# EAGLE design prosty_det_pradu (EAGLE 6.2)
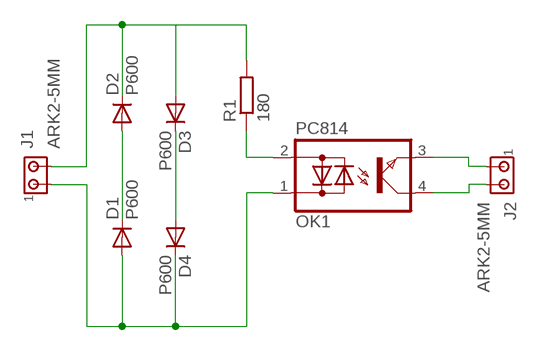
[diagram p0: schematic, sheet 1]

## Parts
D1  P600  [P6-15]
D2  P600  [P6-15]
D3  P600  [P6-15]
D4  P600  [P6-15]
J1  ARK2-5MM  [2PIN-5MM]
J2  ARK2-5MM  [2PIN-5MM]
OK1  PC814  [DIL04]
R1  180  R-EU_0207/7  [0207/7]

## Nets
N$1: D2.C D3.A J1.P$2 R1.2
N$2: D1.C D2.A
N$3: D3.C D4.A
N$5: J2.P$1 OK1.3(E)
N$6: J2.P$2 OK1.4(C)
N$7: D1.A D4.C J1.P$1 OK1.1(AC1)
N$8: OK1.2(AC2) R1.1

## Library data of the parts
D1-D4 = diode:P600: DIODE
J1 J2 = zlacza_futrzak:ARK2: ARK 2
OK1 = optocoupler:PC814: SHARP OPTO COUPLER; OC_FARNELL: 9707662; OC_NEWARK: unknown
R1 = rcl:R-EU_: RESISTOR, European symbol

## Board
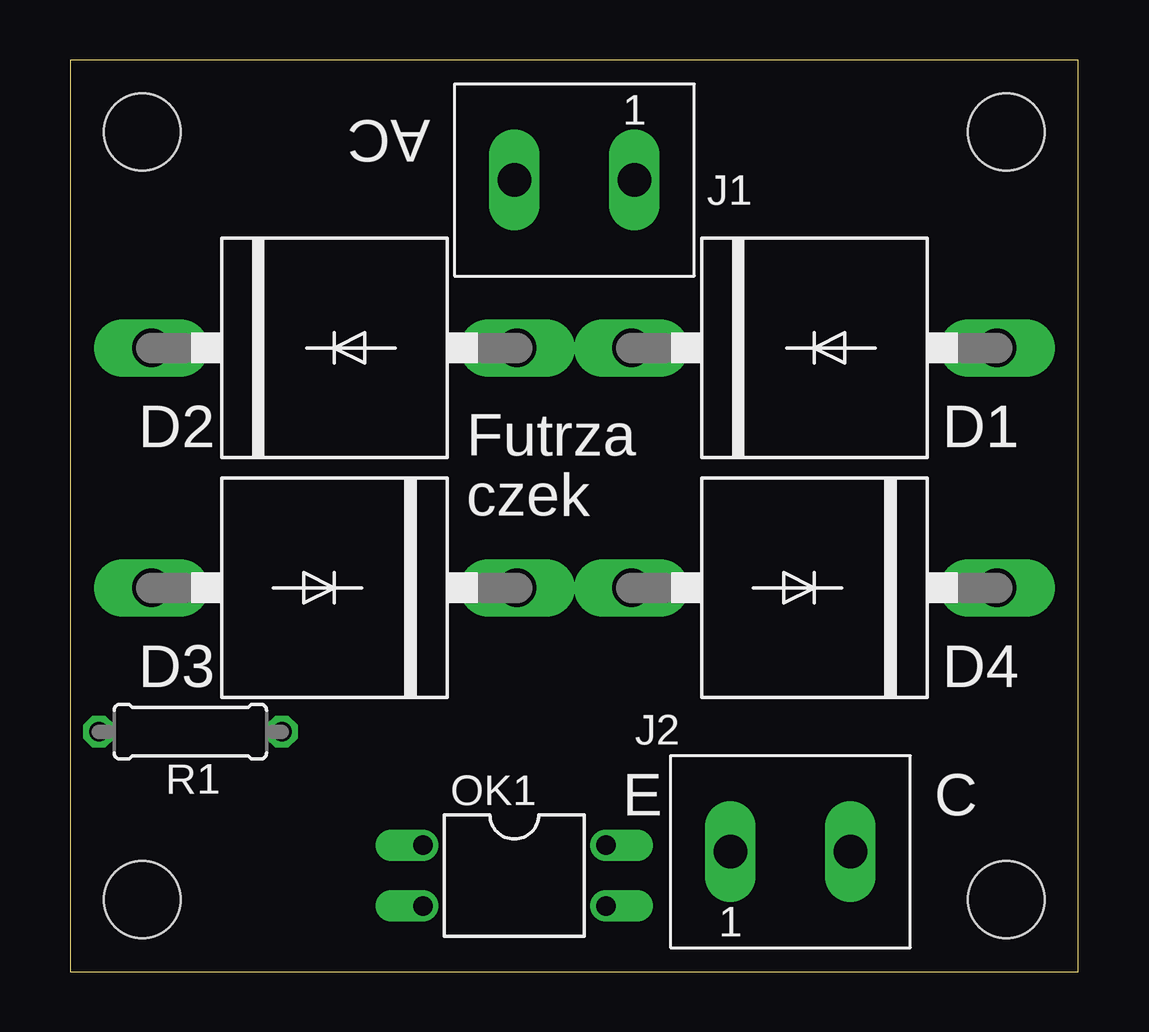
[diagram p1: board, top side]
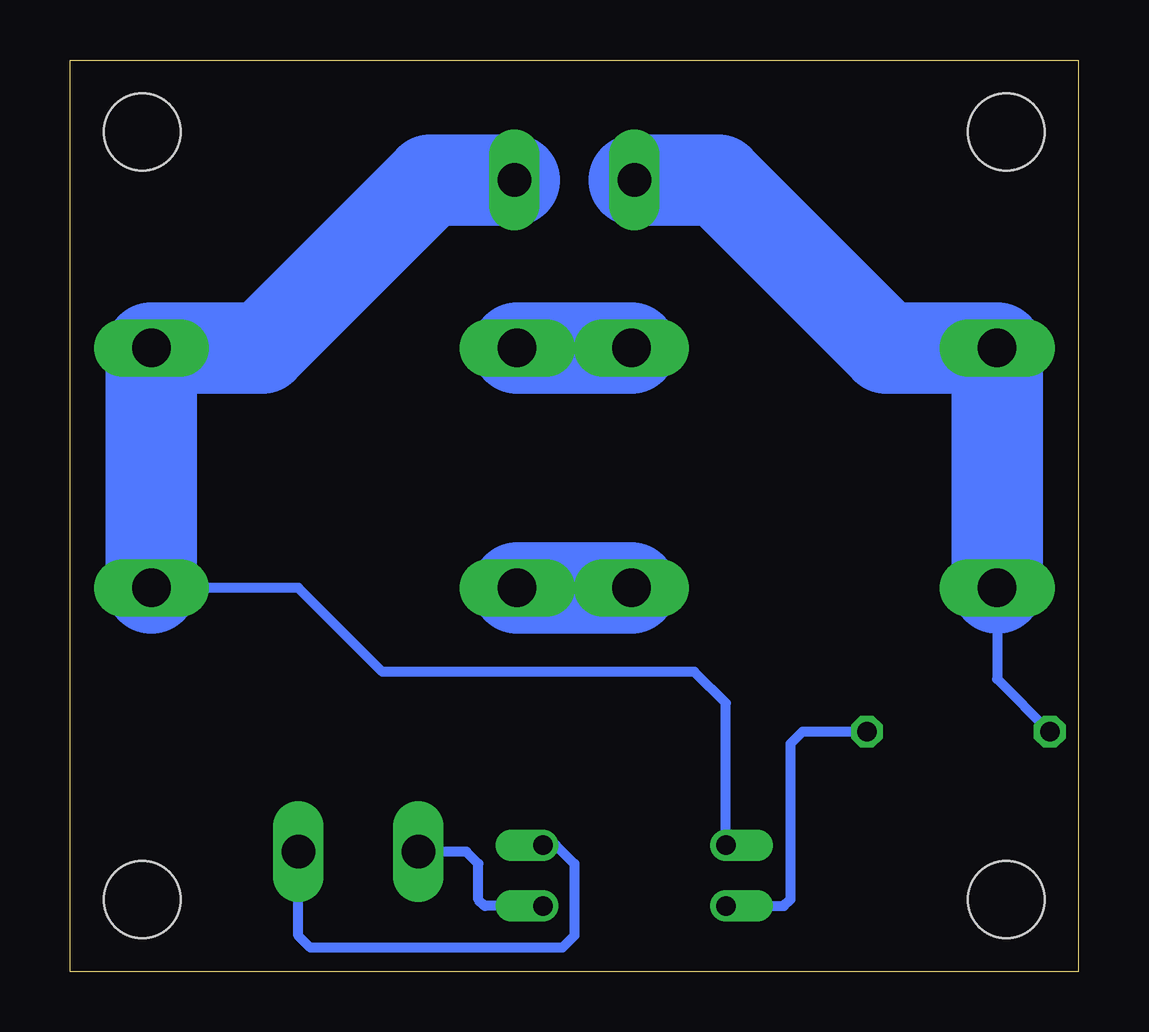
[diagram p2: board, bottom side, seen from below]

Size 42 x 38 mm. Coordinates in mm from the lower left corner, seen from the top.
Outline: 0,0 42,0 42,38 0,38 0,0
Copper layers (1*16): Top 0.035mm / dielectric 1.5mm / Bottom 0.035mm
Design rules: minimum track width 10mil, minimum drill 24mil, track to track 8mil, track to pad 8mil, pad to pad 8mil, via to via 8mil, smd to smd 8mil, copper to edge 40mil, drill to drill 8mil, minimum pad ring 10mil, minimum via ring 8mil, stop-mask expansion 4mil, vias tented up to drill 0mil, thermal gap 10mil
Holes 3.2 mm at 3,35 39,35 3,3 39,3

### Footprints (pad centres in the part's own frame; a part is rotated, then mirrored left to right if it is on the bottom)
P6-15 = drill 1.6 long: A 7.62,0; C -7.62,0
2PIN-5MM = drill 1.4 long: P$1 -2.5,0; P$2 2.5,0
DIL04 = drill 0.813 offset: 1 -1.27,-3.81; 2 1.27,-3.81; 3 1.27,3.81; 4 -1.27,3.81
0207/7 = drill 0.813 octagon: 1 -3.81,0; 2 3.81,0

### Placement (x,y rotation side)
D1  31,26 0 top
D2  11,26 0 top
D3  11,16 180 top
D4  31,16 180 top
J1  21,33 180 top
J2  30,5 0 top
OK1  18.5,4 270 top
R1  5,10 180 top

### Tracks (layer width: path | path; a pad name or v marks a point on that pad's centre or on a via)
N$1
  Bottom 0.406: D3.A 3.38,12.19 R1.2
  Bottom 3.81: J1.P$2 15,33 8,26 D2.C D3.A
N$2
  Bottom 3.81: D2.A D1.C
N$3
  Bottom 3.81: D3.C D4.A
N$5
  Bottom 0.406: OK1.3 24.73,2.73 25,3 25,4.5 25.5,5 J2.P$1
N$6
  Bottom 0.406: OK1.4 21.77,5.27 21,4.5 21,1.5 21.5,1 32,1 32.5,1.5 J2.P$2
N$7
  Bottom 0.406: D4.C 32.5,16 29,12.5 16,12.5 14.69,11.19 OK1.1
  Bottom 3.81: D4.C D1.A 34,26 27,33 J1.P$1
N$8
  Bottom 0.406: R1.1 11.5,10 12,9.5 12,3 12.27,2.73 OK1.2

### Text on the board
tPlace: AC | Futrza | czek | E | C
